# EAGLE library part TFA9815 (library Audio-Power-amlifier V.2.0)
The TFA9815 is a 2-channel power comparator for high-efficiency class D audio amplifier systems. It contains two full-bridge Bridge-Tied Load (BTL) power stages, drive logic, protection control logic and full differential input comparators. By using this power comparator a compact closed-loop self-oscillating digital audio amplifier system or open-loop system can be built. The continuous output power is 2 ´17 W in a full-bridge BTL application. The TFA9815 does not require a heat sink and operates using an asymmetrical supply voltage.
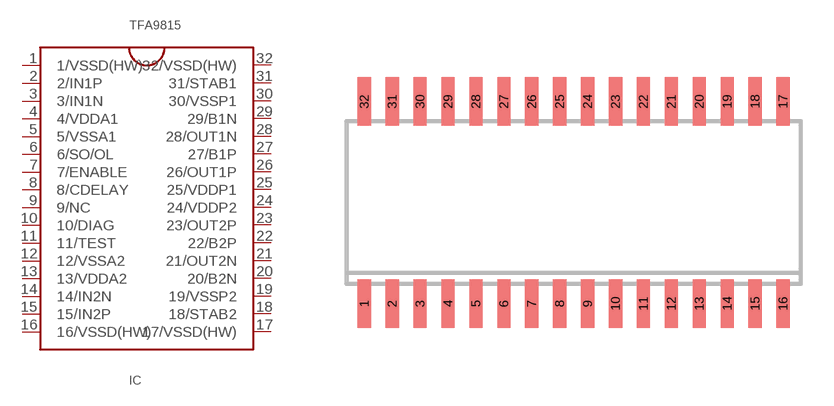
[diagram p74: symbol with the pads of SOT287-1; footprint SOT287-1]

Designator prefix IC

## TFA9815  [SOT287-1]
1  1/VSSD(HW)  pwr
2  2/IN1P  in
3  3/IN1N  in
4  4/VDDA1  pwr
5  5/VSSA1  pwr
6  6/SO/OL
7  7/ENABLE
8  8/CDELAY
9  9/NC  nc
10  10/DIAG
11  11/TEST
12  12/VSSA2  pwr
13  13/VDDA2  pwr
14  14/IN2N  in
15  15/IN2P  in
16  16/VSSD(HW)  pwr
17  17/VSSD(HW)  pwr
18  18/STAB2
19  19/VSSP2  pwr
20  20/B2N
21  21/OUT2N  out
22  22/B2P
23  23/OUT2P  out
24  24/VDDP2  pwr
25  25/VDDP1  pwr
26  26/OUT1P  out
27  27/B1P
28  28/OUT1N  out
29  29/B1N
30  30/VSSP1  pwr
31  31/STAB1
32  32/VSSD(HW)  pwr

## Footprint SOT287-1 (pad centres in mm)
SMALL OUTLINE INTEGRATED CIRCUIT wide body 7.5 mm/JEDEC MO-119AB
smd 0.6 x 2.2: 1 -9.525,-4.6; 2 -8.255,-4.6; 3 -6.985,-4.6; 4 -5.715,-4.6; 5 -4.445,-4.6; 6 -3.175,-4.6; 7 -1.905,-4.6; 8 -0.635,-4.6; 9 0.635,-4.6; 10 1.905,-4.6; 11 3.175,-4.6; 12 4.445,-4.6; 13 5.715,-4.6; 14 6.985,-4.6; 15 8.255,-4.6; 16 9.525,-4.6; 17 9.525,4.6; 18 8.255,4.6; 19 6.985,4.6; 20 5.715,4.6; 21 4.445,4.6; 22 3.175,4.6; 23 1.905,4.6; 24 0.635,4.6; 25 -0.635,4.6; 26 -1.905,4.6; 27 -3.175,4.6; 28 -4.445,4.6; 29 -5.715,4.6; 30 -6.985,4.6; 31 -8.255,4.6; 32 -9.525,4.6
